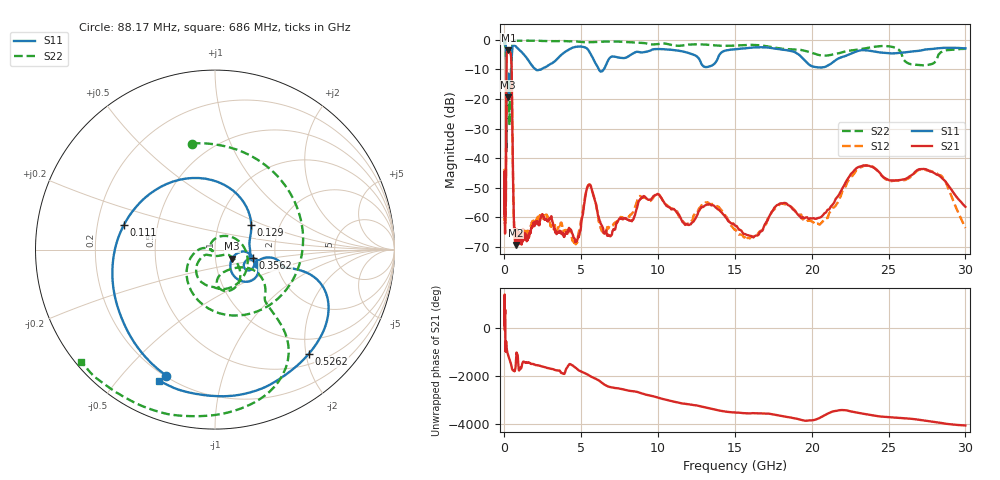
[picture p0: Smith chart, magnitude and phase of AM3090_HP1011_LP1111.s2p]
! Date/Time: Thu, Feb 28, 2019 2:06 PM
! Network Analyzer: Agilent Technologies E8364B Rev: A.07.50.67
! Sweep from 0.010 to 30.000 GHz, 1601 Points, Sweep Type: LOG
! Power Supply: 5.022 V, 0.002 A
# Hz S DB R 50
!freq MagS11 AngS11 MagS21 AngS21 MagS12 AngS12 MagS22 AngS22
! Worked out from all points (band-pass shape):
!   1601 points, 10 MHz to 30 GHz, reference 50 ohm
!   highest |S21| = -3.53 dB at 254.7 MHz (marker M1); lowest = -69.3 dB at 743.2 MHz (marker M2)
!   |S21| within 3 dB of the highest: 133.7 MHz to 442.8 MHz (309.1 MHz wide, 107 % of centre)
!   lowest |S11| = -19.3 dB at 246 MHz (marker M3), VSWR 1.24, Z = 60.2 - j6.16 ohm
!   |S11| at or under -10 dB: 124.6 MHz to 428.5 MHz (303.9 MHz wide, 110 % of centre); 2.036 GHz to 2.39 GHz (353.8 MHz wide, 16 % of centre); 6.145 GHz to 6.463 GHz (318.1 MHz wide, 5.05 % of centre)
!   |S22| runs from -37.8 to -0.2 dB; largest |S21 - S12| = 0.012
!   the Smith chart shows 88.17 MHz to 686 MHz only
!   S11 on the Smith chart (normalised r, x): 88.17 MHz: 0.20, -0.66; 111 MHz: 0.32, +0.12; 129 MHz: 1.43, +0.42; 356.2 MHz: 1.53, -0.15; 526.2 MHz: 0.69, -2.06; 686 MHz: 0.16, -0.65
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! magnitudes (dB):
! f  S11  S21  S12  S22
! 10 MHz  -0.3  -45.4  -46.7  -0.7
! 38.04 MHz  -0.4  -62.1  -57.6  -1.7
! 88.17 MHz  -2.5  -55.2  -53.6  -4.4
! 111 MHz  -5.6  -28.7  -28.6  -6.6
! 129 MHz  -12.2  -8.2  -8.2  -19.2
! 144.7 MHz  -14.1  -5.0  -5.0  -34.4
! 246 MHz  -19.3  -3.5  -3.5  -13.7
! 254.7 MHz  -18.3  -3.5  -3.5  -13.7
! 323.9 MHz  -14.4  -3.6  -3.5  -28.9
! 356.2 MHz  -13.3  -3.9  -3.9  -13.9
! 455.1 MHz  -7.8  -7.8  -7.7  -7.7
! 526.2 MHz  -2.1  -35.1  -35.0  -0.8
! 550.5 MHz  -1.9  -44.0  -43.5  -0.5
! 686 MHz  -2.0  -65.1  -68.0  -0.2
! 743.2 MHz  -2.2  -69.3  -67.0  -0.2
! 2.084 GHz  -10.2  -61.3  -59.8  -0.3
! 4.594 GHz  -2.4  -68.2  -69.3  -0.5
! 5.528 GHz  -4.0  -48.8  -48.9  -0.8
! 7.926 GHz  -6.0  -60.3  -60.1  -0.7
! 15.97 GHz  -2.7  -66.2  -67.1  -1.7
! 23.59 GHz  -3.6  -42.5  -42.4  -2.8
! 30 GHz  -2.9  -56.4  -63.5  -3.0
